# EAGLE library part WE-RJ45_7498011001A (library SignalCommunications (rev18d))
Order Code 7498011001A Design SMD xBase-T 10/100 Base-T Ports 1x1 Application Standard Tab Position Down LED (Left-Right) None EMI Fingers Yes Details see: http://katalog.we-online.de/en/pbs/WE-LAN_RJ45/7498011001A? Updated by Yingchun Shan 2016-08-23 2014 (C) Würth Elektronik
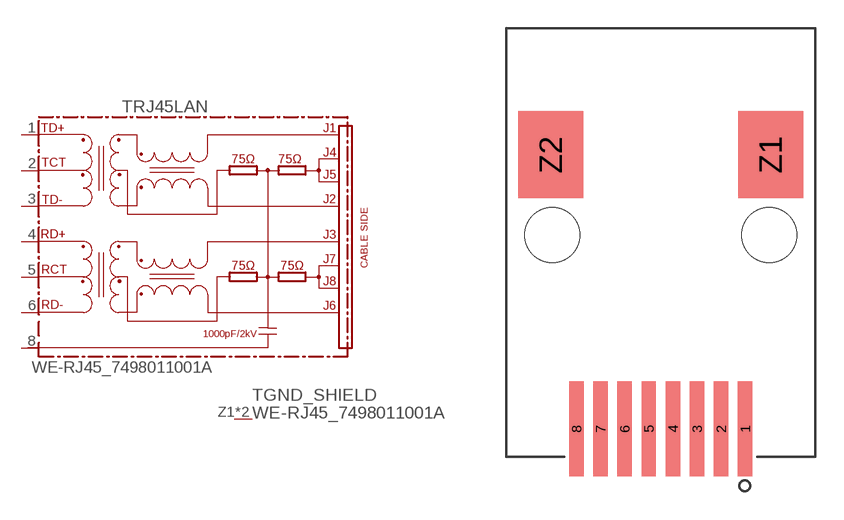
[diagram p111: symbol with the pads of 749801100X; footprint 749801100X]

Designator prefix T; gates RJ45LAN=74990X-THT-10/100-T GND_SHIELD=GND_PIN

## WE-RJ45_7498011001A (COMPANY-URL: http://www.we-online.de; CREATED-BY: Christin Zierenner; CREATED-DATE: AUG 2012; DATASHEET-URL: http://katalog.we-online.de/kataloge/eisos/media/pdf/7498011001A.pdf; MANUFACTURER: Würth Elektronik eiSos GmbH)  [749801100X]
1  RJ45LAN:TD+
2  RJ45LAN:TCT
3  RJ45LAN:TD-
4  RJ45LAN:RD+
5  RJ45LAN:RCT
6  RJ45LAN:RD-
8  RJ45LAN:8
Z1  GND_SHIELD:1  pwr
Z2  GND_SHIELD:1  pwr

## Footprint 749801100X (pad centres in mm)
MAX HEIGHT=13.60mm PORTS----1X1 LED --No
smd 0.76 x 5: 1 4.445,-10.2; 2 3.175,-10.2; 3 1.905,-10.2; 4 0.635,-10.2; 5 -0.635,-10.2; 6 -1.905,-10.2; 7 -3.175,-10.2; 8 -4.445,-10.2
smd 3.42 x 4.58: Z1 5.79,4.24; Z2 -5.79,4.24
hole 2.9 at -5.715,0
hole 2.9 at 5.715,0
